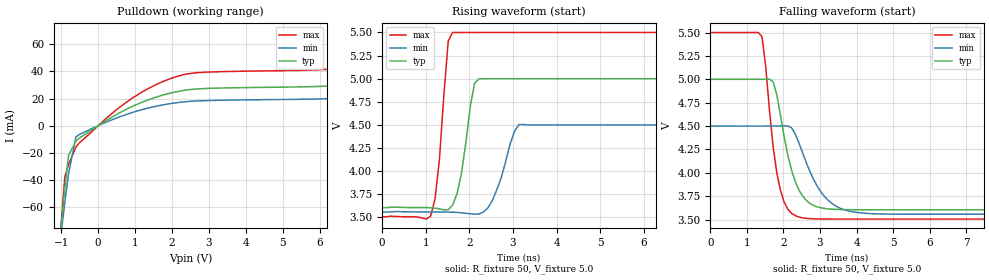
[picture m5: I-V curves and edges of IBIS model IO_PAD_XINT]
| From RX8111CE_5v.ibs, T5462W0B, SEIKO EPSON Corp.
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[Model]   IO_PAD_XINT
Model_type Open_drain
Enable Active-High
Polarity Non-Inverting
Vmeas=2.5
Vref=5.5
Rref=5000
C_comp   2.5p   2.0p   3.0p
[Temperature Range] 25   105   -40
[Voltage Range]   5.0   4.5   5.5
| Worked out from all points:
|   slope of the pulldown table from 0 to 0.75 V, typ, clamps not added: 63 ohm
|   falling waveform, R_fixture 50, V_fixture 5.0: 20-80 % time 478ps typ, 695ps min, 346ps max; typ from 5 V to 3.6 V
|   rising waveform, R_fixture 50, V_fixture 5.0: 20-80 % time 252ps typ, 365ps min, 202ps max; typ from 3.6 V to 5 V
[Pulldown]
-5V       -1.358A    -1.099A    -1.697A
-1.1V     -101.8mA   -101.1mA   -106mA
-900mV    -45.15mA   -55.82mA   -37.2mA
-800mV    -21.58mA   -34.92mA   -28.5mA
-600mV    -11.21mA   -8.18mA    -15.49mA
800mV     12.6mA     8.658mA    18mA
2V        24.33mA    16.48mA    35.1mA
2.7V      27.11mA    18.26mA    39.04mA
7.3V      32.25mA    22.11mA    45.83mA
8.3V      39mA       26.99mA    55.11mA
9.4V      51.58mA    36.18mA    72.08mA
10V       60.61mA    42.84mA    84.12mA
[Falling Waveform]
R_fixture=50
V_fixture=5.0
V_fixture_min=4.5
V_fixture_max=5.5
0s        5V         4.5V       5.5V
1.414ns   5V         4.5V       5.455V
1.717ns   4.974V     4.5V       4.281V
1.818ns   4.837V     4.5V       3.999V
2.02ns    4.385V     4.502V     3.686V
2.323ns   3.907V     4.415V     3.542V
2.626ns   3.704V     4.107V     3.513V
3.03ns    3.626V     3.792V     3.506V
3.737ns   3.606V     3.597V     3.506V
10ns      3.605V     3.557V     3.506V
[Rising Waveform]
R_fixture=50
V_fixture=5.0
V_fixture_min=4.5
V_fixture_max=5.5
0s        3.605V     3.557V     3.506V
1.111ns   3.604V     3.558V     3.512V
1.313ns   3.591V     3.558V     4.122V
1.515ns   3.582V     3.557V     5.406V
1.616ns   3.633V     3.556V     5.5V
1.818ns   3.976V     3.549V     5.5V
2.121ns   4.955V     3.534V     5.5V
2.222ns   4.999V     3.537V     5.5V
3.131ns   5V         4.503V     5.5V
10ns      5V         4.5V       5.5V
[Ramp]
R_load=50
dV/dt_r   8.371E-1/2.450E-10   5.659E-1/3.633E-10   1.197E+0/1.905E-10
dV/dt_f   8.371E-1/4.753E-10   5.659E-1/6.940E-10   1.197E+0/3.434E-10
|[End   IO_PAD_XINT
